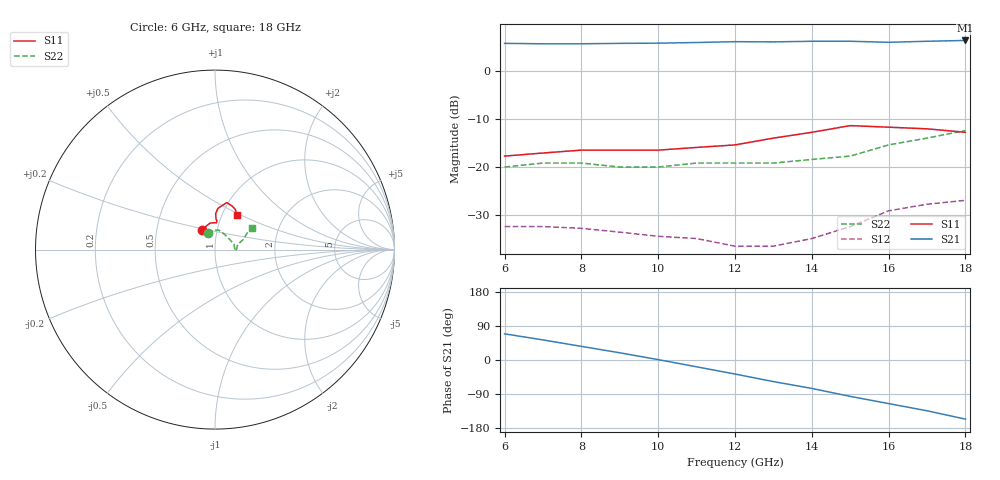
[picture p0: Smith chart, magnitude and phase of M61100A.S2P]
!  MGA-61100 S PARAMETERS
!  Vd=5V  Id=80mA  LAST UPDATED 07-22-92
# ghz s ma r 50
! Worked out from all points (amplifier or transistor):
!   13 points, 6 GHz to 18 GHz, reference 50 ohm
!   highest |S21| = 6.4 dB at 18 GHz (marker M1)
!   |S21| within 3 dB of that: start of sweep to end of sweep
!   unconditionally stable (mu >= 1): start of sweep to end of sweep
!   at 8 GHz: K = 10.97, MAG = 5.8 dB, |S12| = -32.8 dB
!   at 12 GHz: K = 15.86, MAG = 6.3 dB, |S12| = -36.5 dB
!   at 18 GHz: K = 4.76, MAG = 6.9 dB, |S12| = -26.9 dB
6  0.13 123.0  1.94 69.0  0.024 30.0  0.1 114.0
7  0.14 110.0  1.92 53.0  0.024 22.0  0.11 95.0
8  0.15 101.0  1.92 36.0  0.023 13.0  0.11 78.0
9  0.15 91.0  1.94 19.0  0.021 6.0  0.1 57.0
10  0.15 87.0  1.95 1.0  0.019 -5.0  0.1 34.0
11  0.16 86.0  1.98 -18.0  0.018 -14.0  0.11 15.0
12  0.17 88.0  2.02 -37.0  0.015 -14.0  0.11 2.0
13  0.2 89.0  2.01 -57.0  0.015 -28.0  0.11 -3.0
14  0.23 86.0  2.04 -75.0  0.018 -35.0  0.12 1.0
15  0.27 76.0  2.04 -96.0  0.024 -45.0  0.13 13.0
16  0.26 68.0  1.99 -115.0  0.035 -68.0  0.17 20.0
17  0.25 63.0  2.04 -134.0  0.041 -89.0  0.2 27.0
18  0.23 58.0  2.08 -156.0  0.045 -111.0  0.24 30.0
